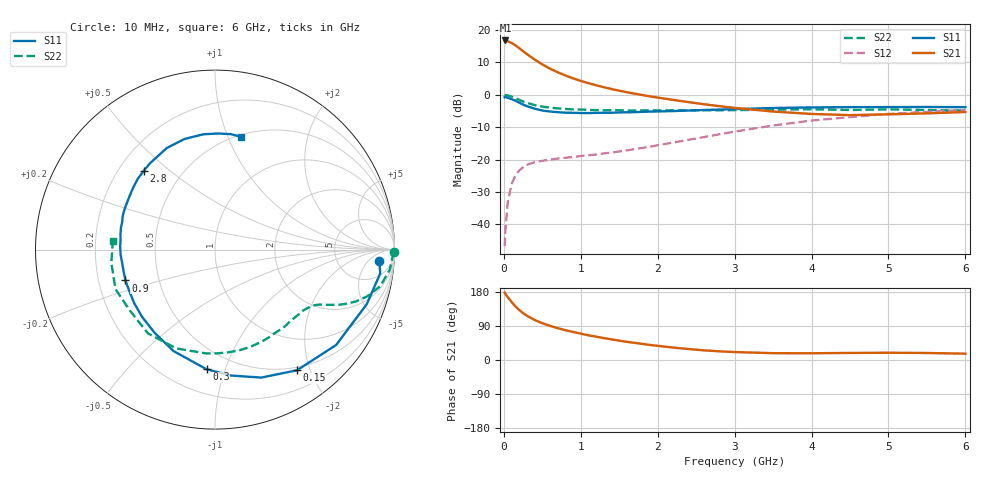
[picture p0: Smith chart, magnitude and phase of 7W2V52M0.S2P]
! Infineon Technologies  Discrete & RF Semiconductors
! BFS17W
! Si NPN RF Bipolar Junction Transistor in SOT323
! VCE = 2.5 V  IC = 2 mA
! Common Emitter S-Parameters:  August  1999
# GHz  S  MA  R  50
!  f  S11  S21  S12  S22
! GHz  MAG  ANG  MAG  ANG  MAG  ANG  MAG  ANG
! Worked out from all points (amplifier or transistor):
!   36 points, 10 MHz to 6 GHz, reference 50 ohm
!   highest |S21| = 16.8 dB at 20 MHz (marker M1)
!   |S21| within 3 dB of that: start of sweep to 233.2 MHz
!   unconditionally stable (mu >= 1): 805.5 MHz to end of sweep
!   at 250 MHz: K = 0.36, MSG = 17.9 dB, |S12| = -22.4 dB
!   at 1.4 GHz: K = 1.33, MAG = 6.4 dB, |S12| = -17.8 dB
!   at 6 GHz: K = 1.10, MAG = -2.3 dB, |S12| = -4.7 dB
!   S11 on the Smith chart (normalised r, x): 10 MHz: 15, -11; 150 MHz: 0.45, -1.80; 300 MHz: 0.36, -0.87; 900 MHz: 0.32, -0.15; 2.8 GHz: 0.30, +0.41; 6 GHz: 0.52, +1.12
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0.01  0.9172 -3.8  6.851 177.9  0.0046 87.4  0.9988 -0.9
0.02  0.9302 -8.2  6.915 174.4  0.0081 85.2  0.9891 -2.6
0.05  0.8987 -19.7  6.728 165.9  0.0215 79.1  0.9801 -6.6
0.1  0.859 -38.2  6.327 153.2  0.0417 69.8  0.9429 -12.5
0.15  0.8129 -55.8  5.813 141.4  0.0567 60.8  0.8885 -17.0
0.2  0.7583 -70.1  5.267 131.8  0.0679 55.0  0.8369 -20.2
0.25  0.7075 -82.7  4.717 123.7  0.0759 49.4  0.7895 -22.5
0.3  0.6685 -94.0  4.257 116.8  0.0829 46.1  0.753 -24.1
0.4  0.6105 -112.3  3.502 105.6  0.0911 41.2  0.6945 -26.3
0.5  0.5725 -126.1  2.952 97.2  0.0957 38.6  0.6592 -27.7
0.6  0.5527 -137.3  2.536 90.0  0.0997 38.0  0.6347 -29.2
0.7  0.5401 -146.6  2.23 84.1  0.1038 38.3  0.6181 -31.0
0.9  0.5278 -161.0  1.796 74.0  0.1097 40.0  0.5958 -34.9
1.1  0.5231 -172.6  1.513 65.2  0.1166 42.8  0.5857 -39.4
1.3  0.5287 177.9  1.312 57.8  0.1246 46.0  0.5781 -44.6
1.6  0.5384 166.5  1.095 47.9  0.1387 50.9  0.5734 -52.5
2.2  0.5611 148.2  0.835 32.8  0.1831 58.8  0.5766 -70.2
2.8  0.5918 132.1  0.669 22.9  0.2452 60.8  0.5783 -89.0
3.5  0.6266 115.4  0.552 18.0  0.3361 57.7  0.5913 -111.3
4.5  0.6457 95.8  0.486 18.6  0.4527 45.9  0.5832 -144.4
5.5  0.6493 82.2  0.517 18.5  0.5478 33.6  0.5823 -172.6
6  0.645 76.9  0.543 16.7  0.5848 27.6  0.5712 175.0
